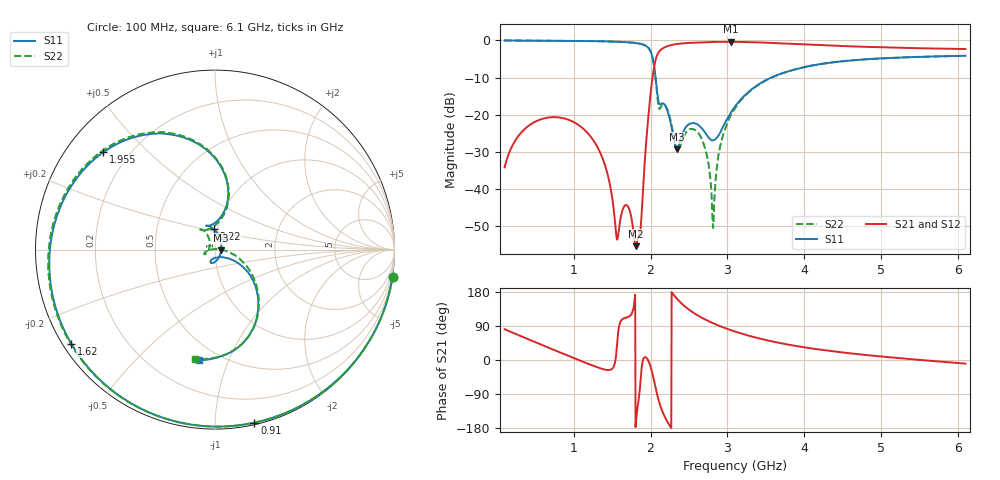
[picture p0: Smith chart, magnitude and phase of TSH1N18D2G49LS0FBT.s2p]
! TSH1N18D2G49LS0FBT  S-PARAMETER MODEL  ( General Type )
! Model Generated by TAIYO YUDEN Corporation (https://www.yuden.co.jp/en/)
! Version 1.0
! TAIYO YUDEN Control No. 20150831
! Copyright(c) 2015 TAIYO YUDEN CO.,LTD. All Rights Reserved.
! Products Name : Multilayer Ceramic Devices
! Characteristics :
!  Passband freq : 2300-2690MHz ( At Passband , Insertion Loss : 1.5dB , VSWR 2.0 ),
!  Attenuation : 35dB min at 1710-1880MHz , Impedance : 50 Ohm ,
!  Case Size : 1.6 x 0.8 / 0.063 x 0.031 [mm/inch] , Thickness : 0.65 / 0.026 [mm/inch]
!  (Conditions: Temperature = 25 degC , DC Bias Current/Voltage = 0A / 0V)
! External Node Assignments :
!  1  o---|-------|---o  2
!  |  HPF  |
! GND o---|-------|---o GND
! Frequency Range : 100MHz  -  6.1GHz  [ 1201 STEP ]
# MHZ S RI R 50
! Freq[MHz].  S11 Real  S11 Imag  S21 Real  S21 Imag  S12 Real  S12 Imag  S22 Real  S22 Imag
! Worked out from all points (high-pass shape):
!   1201 points, 100 MHz to 6.1 GHz, reference 50 ohm
!   highest |S21| = -0.35 dB at 3.045 GHz (marker M1); lowest = -55.4 dB at 1.81 GHz (marker M2)
!   |S21| within 3 dB of the highest: 2.1 GHz to end of sweep
!   lowest |S11| = -29.3 dB at 2.34 GHz (marker M3), VSWR 1.07, Z = 53.5 - j0.389 ohm
!   |S11| at or under -10 dB: 2.066 GHz to 3.57 GHz (1.504 GHz wide, 53.4 % of centre)
!   |S22| runs from -50.5 to 0.0 dB; largest |S21 - S12| = 0.0024
!   S11 on the Smith chart (normalised r, x): 100 MHz: -0, -13; 910 MHz: 0.01, -1.25; 1.62 GHz: 0.02, -0.30; 1.955 GHz: 0.11, +0.37; 2.22 GHz: 0.96, +0.22; 6.1 GHz: 0.39, -0.79
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100  0.9893 -0.1506  0.003 0.0193  0.00297 0.0193  0.9892 -0.1525
415  0.8112 -0.581  0.0417 0.0577  0.0417 0.0578  0.8057 -0.5891
910  0.2198 -0.964  0.0849 0.0189  0.0848 0.0188  0.1882 -0.9705
1100  -0.059 -0.9832  0.0679 -0.00361  0.0678 -0.00373  -0.1019 -0.9793
1395  -0.5007 -0.8359  0.0206 -0.00956  0.0206 -0.00961  -0.5482 -0.8054
1560  -0.7284 -0.63  0.00187 0.0011  0.00187 0.00107  -0.7656 -0.5847
1620  -0.8004 -0.5247  -0.00115 0.00438  -0.00116 0.00436  -0.8312 -0.4755
1810  -0.9222 -0.0317  -0.00164 -0.000424  -0.00165 -0.000437  -0.9248 0.0144
1870  -0.8794 0.1901  0.0017 -0.00232  0.00172 -0.0023  -0.8734 0.2287
1955  -0.6221 0.5429  0.0597 0.00405  0.0597 0.00399  -0.6089 0.5631
2040  0.00811 0.4991  0.2627 -0.3029  0.2627 -0.3029  0.0177 0.4926
2100  0.0106 0.1577  -0.1427 -0.6637  -0.1427 -0.6639  0.000417 0.1352
2220  -0.00549 0.113  -0.802 -0.2425  -0.8022 -0.2423  -0.0582 0.1014
2340  0.034 -0.00363  -0.855 0.2678  -0.855 0.2681  -0.0302 0.0165
2635  -0.0256 -0.0661  -0.4024 0.8514  -0.4027 0.8518  -0.053 -0.0129
2815  0.00823 -0.0443  -0.1166 0.948  -0.1166 0.9481  9.66e-05 0.00299
2905  0.0385 -0.0417  0.0105 0.9585  0.0107 0.9587  0.0369 -0.000661
3045  0.0908 -0.0554  0.1859 0.9421  0.1859 0.9419  0.0955 -0.0226
3100  0.1119 -0.0643  0.2468 0.9267  0.2469 0.927  0.1169 -0.0355
4100  0.2284 -0.3981  0.755 0.4444  0.7553 0.4444  0.2292 -0.3973
5100  0.08 -0.5754  0.7975 0.1042  0.7975 0.1043  0.0803 -0.5746
6100  -0.0896 -0.6167  0.757 -0.1279  0.7581 -0.1291  -0.1108 -0.6101
